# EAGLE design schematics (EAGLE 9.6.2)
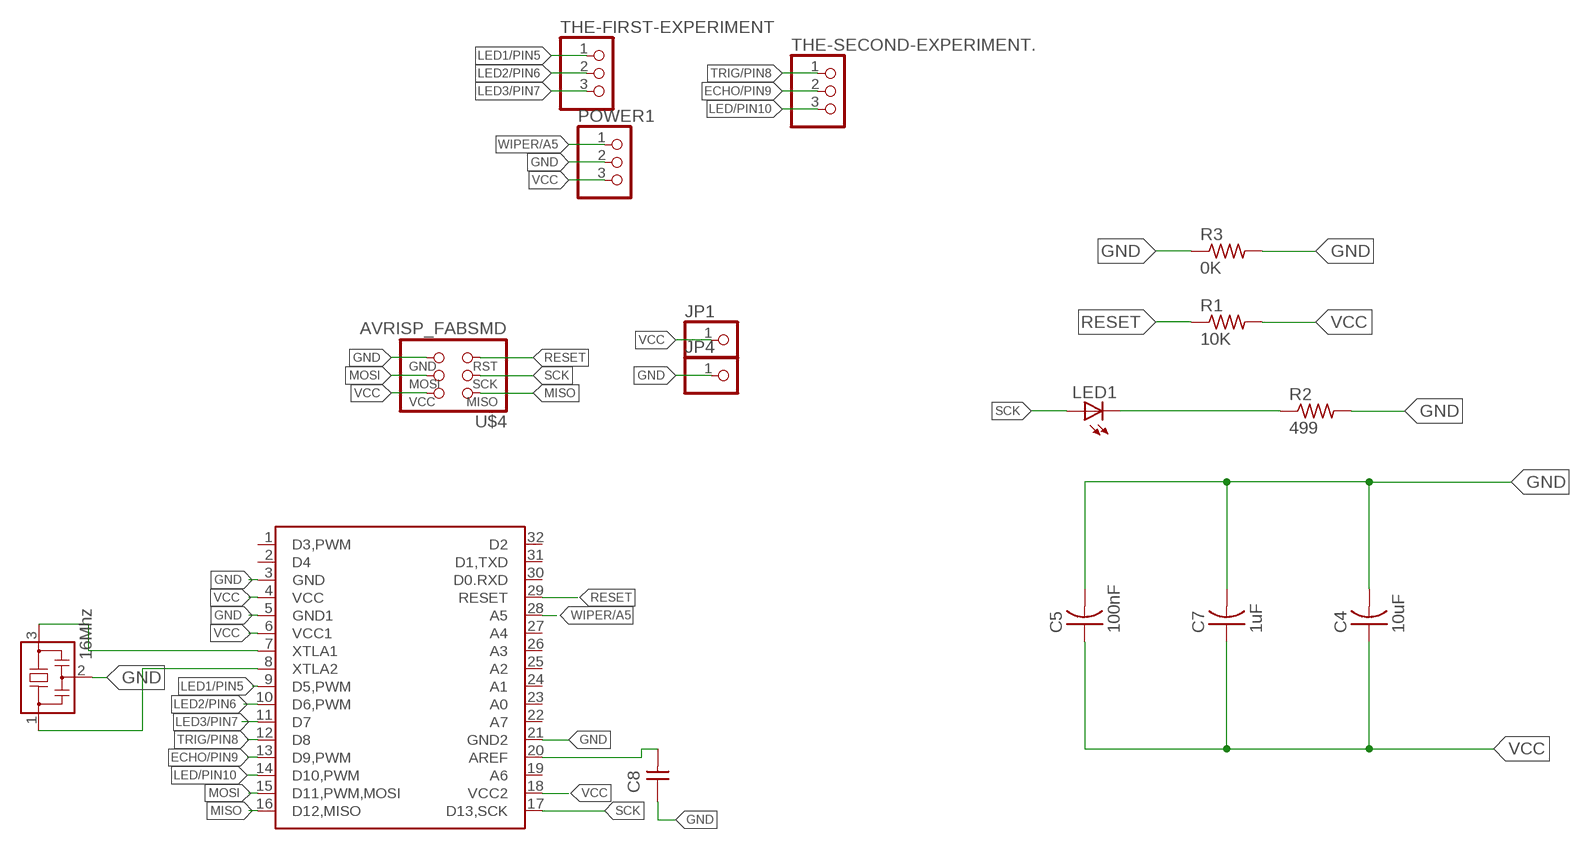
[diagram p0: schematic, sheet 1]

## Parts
C4  10uF  CAP-US1206FAB  [C1206FAB]
C5  100nF  CAP-US1206FAB  [C1206FAB]
C7  1uF  CAP-US1206FAB  [C1206FAB]
C8  CAP-UNPOLARIZEDFAB  [C1206FAB]
JP1  PINHD-1X1CB  [1X01-CLEANBIG]
JP4  PINHD-1X1CB  [1X01-CLEANBIG]
LED1  LEDSMT1206  [1206]
POWER1  PINHD-1X3CB  [1X03-CLEANBIG]
R1  10K  RES-US1206FAB  [R1206FAB]
R2  499  MCS1632R050FER  [RES_1206]
R3  0K  RES-US1206FAB  [R1206FAB]
RESONATOR1  16Mhz  RESONATOR  [EFOBM]
THE-FIRST-EXPERIMENT  PINHD-1X3CB  [1X03-CLEANBIG]
THE-SECOND-EXPERIMENT.  PINHD-1X3CB  [1X03-CLEANBIG]
U$1  ATMEGA328P_TQFP_FAB.03  [QFP80P900X900X120-32L]
U$4  AVRISP_FABSMD  [2X03SMD]

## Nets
ECHO/PIN9: THE-SECOND-EXPERIMENT..2 U$1.13(D9,PWM)
GND: C4.2 C5.2 C7.2 C8.1 JP4.1 POWER1.2 R2.2 R3.1 R3.2 RESONATOR1.2 U$1.3(GND) U$1.5(GND1) U$1.21(GND2) U$4.6(GND)
LED1/PIN5: THE-FIRST-EXPERIMENT.1 U$1.9(D5,PWM)
LED2/PIN6: THE-FIRST-EXPERIMENT.2 U$1.10(D6,PWM)
LED3/PIN7: THE-FIRST-EXPERIMENT.3 U$1.11(D7)
LED/PIN10: THE-SECOND-EXPERIMENT..3 U$1.14(D10,PWM)
MISO: U$1.16(D12,MISO) U$4.1(MISO)
MOSI: U$1.15(D11,PWM,MOSI) U$4.4(MOSI)
N$1: RESONATOR1.3 U$1.7(XTLA1)
N$5: RESONATOR1.1 U$1.8(XTLA2)
N$7: C8.2 U$1.20(AREF)
N$8: LED1.C R2.1
RESET: R1.1 U$1.29(RESET) U$4.5(RST)
SCK: LED1.A U$1.17(D13,SCK) U$4.3(SCK)
TRIG/PIN8: THE-SECOND-EXPERIMENT..1 U$1.12(D8)
VCC: C4.1 C5.1 C7.1 JP1.1 POWER1.3 R1.2 U$1.4(VCC) U$1.6(VCC1) U$1.18(VCC2) U$4.2(VCC)
WIPER/A5: POWER1.1 U$1.28(A5)
Unconnected: U$1.1(D3,PWM) U$1.2(D4) U$1.19(A6) U$1.22(A7) U$1.23(A0) U$1.24(A1) U$1.25(A2) U$1.26(A3) U$1.27(A4) U$1.30(D0.RXD) U$1.31(D1,TXD) U$1.32(D2)

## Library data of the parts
C4 C5 C7 = fab:CAP-US
C8 = fab:CAP-UNPOLARIZED
JP1 JP4 = adafruit:PINHD-1X1: Pin header 1x1 for 0.1" spacing
LED1 = adafruit:LED: LED
POWER1 THE-FIRST-EXPERIMENT THE-SECOND-EXPERIMENT. = adafruit:PINHD-1X3: PIN HEADER
R1 R3 = fab:RES-US: Resistor (US Symbol)
R2 = Resistor_Capacitor:MCS1632R050FER: RES 0.05 OHM 1% 1W 1632; CREATED_BY: PCBLayout.com; DIGIKEY_PART_NUMBER: MCS1632R050FERTR-ND; MANUFACTURER: Ohmite; MPN: MCS1632R050FER; PACKAGE: SMD 1206
RESONATOR1 = fab:RESONATOR
U$1 = fablab:ATMEGA328P_TQFP_FAB.03
U$4 = fablab (1):AVRISP_FAB

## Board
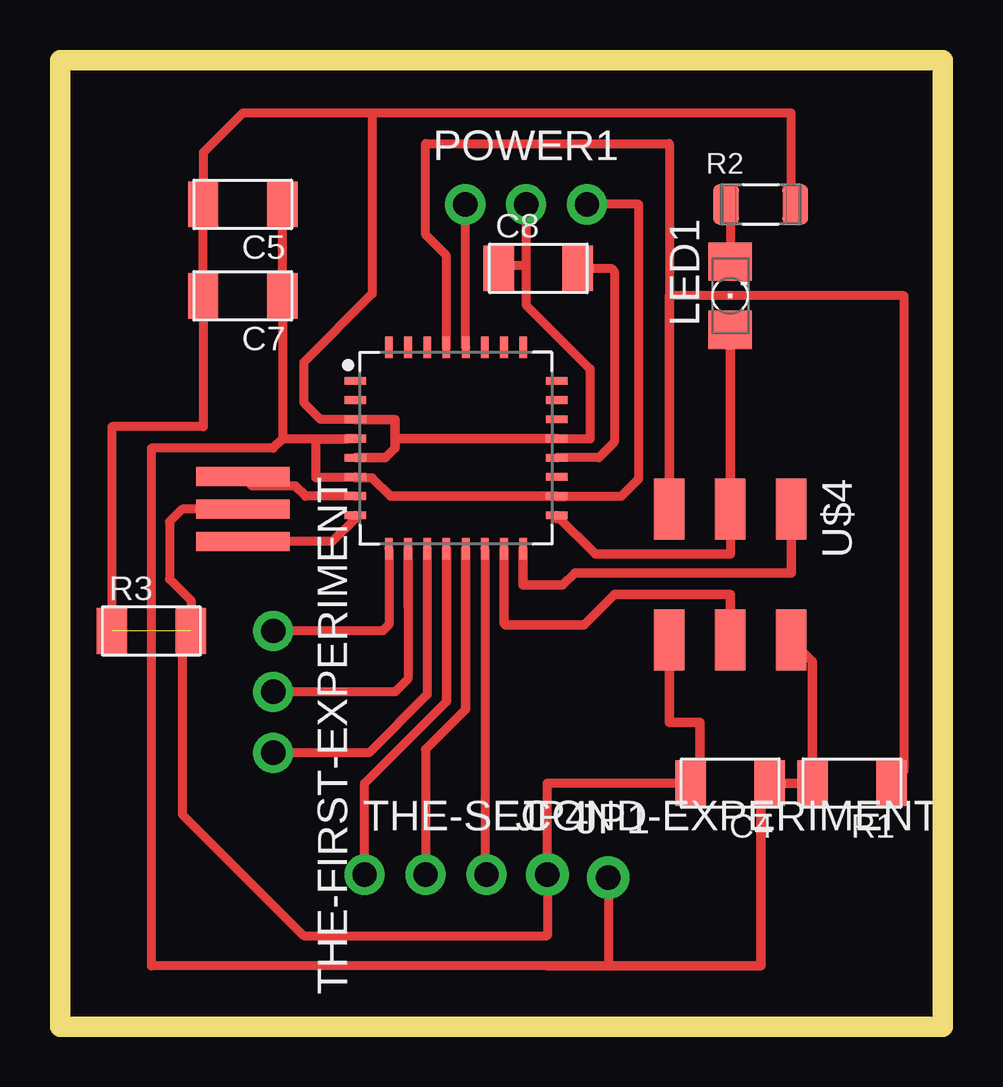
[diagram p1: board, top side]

Size 36.81 x 40.31 mm. Coordinates in mm from the lower left corner, seen from the top.
Outline: 0,0 36.81,0 36.81,40.31 0,40.31 0,0
Copper layers (1*16): Top 0.035mm / dielectric 1.5mm / Bottom 0.035mm
Design rules "default *": minimum track width 0.38mm, minimum drill 0.35mm, track to track 0.38mm, track to pad 0.38mm, pad to pad 0.38mm, via to via 0.38mm, smd to smd 0.38mm, copper to edge 40mil, drill to drill 6mil, minimum pad ring 10mil, minimum via ring 8mil, stop-mask expansion 4mil, vias tented up to drill 0mil, thermal gap 10mil

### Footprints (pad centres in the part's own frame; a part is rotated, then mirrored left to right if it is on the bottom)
C1206FAB = smd 1.27 x 1.905: 1 -1.651,0; 2 1.651,0
1X01-CLEANBIG = drill 1.016 pad 1.778: 1 0,0
1206 = smd 1.6 x 1.803: A -1.422,0; C 1.422,0
1X03-CLEANBIG = drill 1.016 pad 1.676: 1 -2.54,0; 2 0,0; 3 2.54,0
R1206FAB = smd 1.27 x 1.905: 1 -1.651,0; 2 1.651,0
RES_1206 = smd 1.08 x 1.68: 1 -1.445,0; 2 1.445,0
EFOBM = smd 0.8 x 3.9: 1 -1.35,0; 2 0,0; 3 1.35,0
QFP80P900X900X120-32L = smd 0.906 x 0.32: 1 -4.197,2.8; 2 -4.197,2; 3 -4.197,1.2; 4 -4.197,0.4; 5 -4.197,-0.4; 6 -4.197,-1.2; 7 -4.197,-2; 8 -4.197,-2.8; 17 4.197,-2.8; 18 4.197,-2; 19 4.197,-1.2; 20 4.197,-0.4; 21 4.197,0.4; 22 4.197,1.2; 23 4.197,2; 24 4.197,2.8 | smd 0.32 x 0.906: 9 -2.8,-4.197; 10 -2,-4.197; 11 -1.2,-4.197; 12 -0.4,-4.197; 13 0.4,-4.197; 14 1.2,-4.197; 15 2,-4.197; 16 2.8,-4.197; 25 2.8,4.197; 26 2,4.197; 27 1.2,4.197; 28 0.4,4.197; 29 -0.4,4.197; 30 -1.2,4.197; 31 -2,4.197; 32 -2.8,4.197
2X03SMD = smd 2.54 x 1.27: 1 -2.54,2.54; 2 2.92,2.54; 3 -2.54,0; 4 2.92,0; 5 -2.54,-2.54; 6 2.92,-2.54

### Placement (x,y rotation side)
C4  27.94,10.16 180 top
C5  7.62,34.29 180 top
C7  7.62,30.48 180 top
C8  19.94,31.62 0 top
JP1  22.86,6.22 0 top
JP4  20.32,6.35 0 top
LED1  27.94,30.48 90 top
POWER1  19.43,34.29 0 top
R1  33.02,10.16 180 top
R2  29.21,34.29 0 top
R3  3.81,16.51 0 top
RESONATOR1  7.62,21.59 90 top
THE-FIRST-EXPERIMENT  8.89,13.97 270 top
THE-SECOND-EXPERIMENT.  15.24,6.35 0 top
U$1  16.51,24.13 0 top
U$4  27.94,19.05 270 top

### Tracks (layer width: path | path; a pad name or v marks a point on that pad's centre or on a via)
ECHO/PIN9
  Top 0.38: 15.24,11.57 THE-SECOND-EXPERIMENT..2
  Top 0.4: 15.24,11.57 16.91,13.24 U$1.13
GND  (1 unrouted)
  Top 0.38: POWER1.2 19.43,31.75 | 19.43,31.75 19.43,30.1 22.1,27.43 22.1,24.51 20.73,24.51 U$1.21 | C8.1 18.41,31.75 19.43,31.75 | 26.67,9.78 C4.2 20.32,10.16 JP4.1 20.32,3.81 10.16,3.81 5.1,8.87 5.1,16.15 R3.2 5.46,17.78 4.57,18.67 4.57,21.06 5.1,21.59 RESONATOR1.2 | R2.2 30.48,34.47 30.48,38.1 12.7,38.1 | U$1.3 10.86,25.33 10.16,26.03 10.16,27.7 13.02,30.56 13.02,38.1 7.62,38.1 5.97,36.45 C5.2 C7.2 5.97,25.02 2.16,25.02 R3.1
  Top 0.4: U$4.6 25.4,12.7 26.67,12.7 26.67,10.54 C4.2 | U$1.5 13.57,23.73 13.97,24.13 13.97,24.64 | U$1.3 13.97,25.33 13.97,24.64 | 13.97,24.64 14.08,24.53 U$1.21
LED1/PIN5
  Top 0.38: U$1.9 13.71,16.77 13.45,16.51 THE-FIRST-EXPERIMENT.1
LED2/PIN6
  Top 0.38: 14.51,17.78 14.51,14.51 13.97,13.97 THE-FIRST-EXPERIMENT.2
  Top 0.4: U$1.10 14.51,17.78 14.51,17.53
LED3/PIN7
  Top 0.38: THE-FIRST-EXPERIMENT.3 12.88,11.43 15.31,13.86 U$1.11
LED/PIN10
  Top 0.38: U$1.14 17.71,6.42 THE-SECOND-EXPERIMENT..3
MISO
  Top 0.4: U$1.16 19.31,18.41 20.96,18.41 21.46,18.92 30.48,18.92 U$4.1
MOSI
  Top 0.4: U$4.4 27.94,18.03 23.11,18.03 21.84,16.76 18.58,16.76 18.51,16.83 U$1.15
N$1
  Top 0.38: RESONATOR1.3 8,22.56 9.81,22.56 10.24,22.13 U$1.7
  Top 0.4: RESONATOR1.3 7.7,22.86
N$5
  Top 0.38: U$1.8 12.31,21.2 11.35,20.24 7.7,20.24
  Top 0.4: 7.7,20.24 RESONATOR1.1
N$7
  Top 0.38: C8.2 22.99,31.62 23.11,31.5 23.11,24.38 22.46,23.73 U$1.20
N$8
  Top 0.38: R2.1 27.94,34.12 LED1.C
RESET
  Top 0.38: R1.1 35.18,10.67 35.18,30.48 25.4,30.48 25.4,36.83 15.24,36.83 15.24,33.02 16.11,32.15 U$1.29
  Top 0.4: U$4.5 25.4,30.48
SCK
  Top 0.38: U$4.3 27.94,19.72
  Top 0.4: LED1.A U$4.3 | 20.71,21.2 U$1.17 22.31,19.72 27.94,19.72
TRIG/PIN8
  Top 0.38: THE-SECOND-EXPERIMENT..1 12.7,10.16
  Top 0.4: U$1.12 16.11,13.57 12.7,10.16
VCC
  Top 0.38: C5.1 C7.1 9.27,24.51 | 13.01,22.89 13,22.9 12.34,22.9 U$1.6 12.28,22.9 10.67,22.9 10.67,24.51 | 20.32,2.54 3.81,2.54 3.81,24.13 8.89,24.13 9.27,24.51 | 21.03,22.1 20.74,22.1 U$1.18 23.4,22.13 24.13,22.86 24.13,34.29 POWER1.3 | 11.43,24.51 9.27,24.51 | JP1.1 22.86,2.54
  Top 0.4: 20.32,2.54 22.86,2.54 29.21,2.54 29.21,9.78 C4.1 R1.2 31.37,15.24 U$4.2 | U$1.18 13.77,22.13 13.01,22.89 | U$1.4 11.98,24.53 11.96,24.51 11.43,24.51 10.67,24.51
WIPER/A5
  Top 0.38: U$1.28 16.91,34.27 POWER1.1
